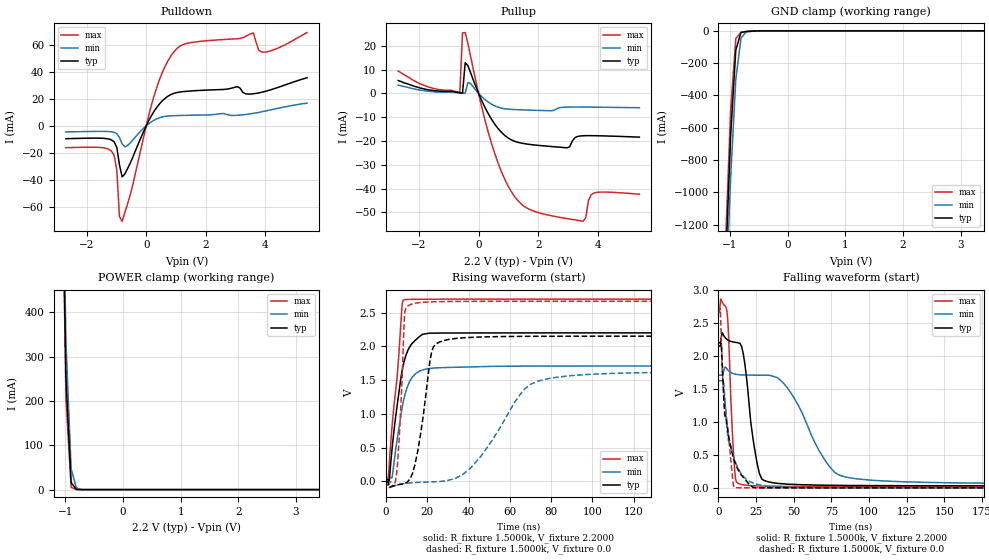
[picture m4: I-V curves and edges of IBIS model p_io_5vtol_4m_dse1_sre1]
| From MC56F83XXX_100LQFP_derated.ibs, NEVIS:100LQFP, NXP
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[Model] p_io_5vtol_4m_dse1_sre1
|   Model p_io_5vtol_4m_dse1_sre1
| Library cells for typ/min/max conditions are connected as defined below:
|  pad - External Pad
|  ipp_do - Core Input
|  ipp_obe - Output Buffer Enable
|  esd_boost - vdd_s_3v
|  esd_bus - vdd_s_3v
|  ipp_ame - vss_s_lv
|  ipp_dse - vdd_s_lv
|  ipp_ina40a_5vtol - NC
|  ipp_ina40b_5vtol - NC
|  ipp_ina_5vtol - NC
|  ipp_ina_mux_3v - NC
|  ipp_ind - NC
|  ipp_ind_3v - NC
|  ipp_pue - vss_s_lv
|  ipp_sre - vdd_s_lv
|  tie_3v - vdd_s_3v
|  tie_hi - vdd_s_lv
|  vbuf_3v - vdd_s_3v
|  vdd_bulk_lv - vdd_s_lv
|  vdd_s_3v - vdd_s_3v
|  vdd_s_lv - vdd_s_lv
|  vss_bulk - vss_s_3v
|  vss_s_3v - vss_s_3v
|  vss_s_lv - vss_s_lv
| All other pins connected to ground
Model_type I/O
Polarity   Non-Inverting
Enable   Active-High
Vinl =   0.7700V
Vinh =   1.5400V
Vmeas =  1.1000V
Cref =   25.0000pF
Rref =   1.0000k
Vref =   0.0V
C_comp   2.5897pF   2.5141pF   2.6932pF
[Temperature Range]   25.0000   0.1250k   -40.0000
[Voltage Range]   2.2000V   1.7100V   2.7000V
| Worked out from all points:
|   slope of the pulldown table from 0 to 0.33 V, typ, clamps not added: 25.7 ohm
|   slope of the pullup table from 0 to 0.33 V, typ, clamps not added: 38.3 ohm
|   GND clamp passes 1 mA (typ) near -0.56 V on its own axis
|   POWER clamp passes 1 mA (typ) near -0.81 V on its own axis
|   rising waveform, R_fixture 1.5000k, V_fixture 2.2000: 20-80 % time 5.84ns typ, 5.78ns min, 4.56ns max; typ from 0.031 V to 2.2 V
|   rising waveform, R_fixture 1.5000k, V_fixture 0.0: 20-80 % time 5.78ns typ, 20.7ns min, 2.31ns max; typ from 0 V to 2.15 V
|   falling waveform, R_fixture 1.5000k, V_fixture 2.2000: 20-80 % time 6.8ns typ, 21.8ns min, 2.96ns max; typ from 2.2 V to 0.031 V
|   falling waveform, R_fixture 1.5000k, V_fixture 0.0: 20-80 % time 7.59ns typ, 8.09ns min, 5.81ns max; typ from 2.15 V to 0 V
[Pulldown]
|Voltage   I(typ)   I(min)   I(max)
-2.7V     -9.58mA    -4.57mA    -16.24mA
-1.17V    -10.45mA   -4.486mA   -18.73mA
-990mV    -15.98mA   -5.899mA   -32.6mA
-900mV    -28.96mA   -8.727mA   -67.1mA
-810mV    -37.86mA   -13.49mA   -70.68mA
270mV     10.92mA    4.186mA    22.64mA
990mV     24.34mA    7.49mA     56.19mA
3.06V     28.9mA     7.71mA     64.33mA
3.6V      23.63mA    9.2mA      68.56mA
3.78V     24.28mA    9.8mA      55.81mA
4.05V     25.71mA    11.1mA     54.67mA
5.4V      35.5mA     16.7mA     68.9mA
[Pullup]
|Voltage   I(typ)   I(min)   I(max)
-2.7V     5.4mA      3.5mA      9.4mA
-630mV    252.5uA    218.2uA    372uA
-540mV    133.6uA    121.1uA    25.42mA
-450mV    12.88mA    56.63uA    25.55mA
-270mV    8.722mA    4.155mA    15.59mA
540mV     -12.86mA   -5.202mA   -25.17mA
990mV     -18.7mA    -6.605mA   -38.86mA
1.44V     -20.88mA   -6.905mA   -46.53mA
2.97V     -22.84mA   -5.75mA    -52.58mA
3.51V     -17.79mA   -5.732mA   -53.71mA
3.87V     -17.76mA   -5.78mA    -41.87mA
5.4V      -18.36mA   -6.02mA    -42.31mA
[GND_clamp]
|Voltage   I(typ)   I(min)   I(max)
-2.7V     -20.35A    -20.38A    -20.37A
-1.08V    -1.486A    -1.737A    -1.339A
-990mV    -654.8mA   -915.7mA   -496.6mA
-900mV    -120.3mA   -300.6mA   -47.98mA
-810mV    -10.43mA   -45.61mA   -9.206mA
-720mV    -3.577mA   -6.172mA   -6.342mA
-540mV    -682.6uA   -563.7uA   -1.265mA
5.4V      0A         0A         0A
[POWER_clamp]
|Voltage   I(typ)   I(min)   I(max)
-2.7V     20.23A     19.96A     20.45A
-1.08V    950.5mA    990.2mA    948mA
-990mV    252.7mA    333.8mA    206.6mA
-900mV    16.05mA    47.59mA    5.278mA
-810mV    508.3uA    3.841mA    61.17uA
-720mV    15.33uA    281.3uA    694.4nA
-630mV    461.8nA    20.43uA    7.955nA
5.4V      0A         0A         0A
[Ramp]
| variable   typ   min   max
dV/dt_r  0.6016/24.4085n   0.2055/56.3670n   1.0880/10.0620n
dV/dt_f  0.7284/40.9818n   0.2179/77.6681n   1.2636/15.3351n
R_load = 50.0000
[Rising Waveform]
R_fixture= 1.5000k
V_fixture= 2.2000
V_fixture_min= 1.7100
V_fixture_max= 2.7000
|time   V(typ)   V(min)   V(max)
0s        31.17mV    60.03mV    18.84mV
899.9ps   31.66mV    60.02mV    -22.79mV
1.51ns    13.16mV    60.44mV    267.9mV
2.898ns   495.8mV    62.89mV    830.2mV
5.303ns   1.116V     615.1mV    1.54V
7.252ns   1.558V     1.004V     2.424V
8.289ns   1.724V     1.181V     2.687V
14.25ns   2.094V     1.596V     2.698V
24.37ns   2.196V     1.682V     2.699V
250ns     2.2V       1.71V      2.7V
[Rising Waveform]
R_fixture= 1.5000k
V_fixture= 0.0
V_fixture_min= 0.0
V_fixture_max= 0.0
|time   V(typ)   V(min)   V(max)
0s        554.5pV    116.9nV    15.42pV
4.607ns   -56.99mV   -58.21mV   18.73mV
6.434ns   -45.92mV   -44.25mV   696mV
8.886ns   -28.72mV   -31.27mV   2.436V
12.57ns   105.7mV    -20.07mV   2.628V
22.09ns   1.925V     -8.013mV   2.66V
27.79ns   2.085V     3.953mV    2.664V
40.95ns   2.133V     198.4mV    2.667V
78.42ns   2.15V      1.521V     2.668V
250ns     2.151V     1.626V     2.668V
[Falling Waveform]
R_fixture= 1.5000k
V_fixture= 2.2000
V_fixture_min= 1.7100
V_fixture_max= 2.7000
|time   V(typ)   V(min)   V(max)
0s        2.2V       1.71V      2.7V
5.586ns   2.253V     1.806V     2.691V
10.58ns   2.21V      1.729V     321.7mV
13.08ns   2.201V     1.719V     68.43mV
17.53ns   1.881V     1.712V     42.81mV
25.7ns    370.6mV    1.71V      29.35mV
31.91ns   98.53mV    1.71V      25.6mV
46.04ns   55.8mV     1.51V      21.78mV
80.6ns    37.23mV    188.8mV    19.29mV
250ns     31.22mV    63.37mV    18.84mV
[Falling Waveform]
R_fixture= 1.5000k
V_fixture= 0.0
V_fixture_min= 0.0
V_fixture_max= 0.0
|time   V(typ)   V(min)   V(max)
0s        2.151V     1.626V     2.668V
1.232ns   2.151V     1.626V     2.692V
2.001ns   2.125V     1.626V     2.105V
3.213ns   1.464V     1.635V     1.524V
4.117ns   1.127V     1.391V     1.345V
6.31ns    851mV      756.6mV    860.5mV
9.298ns   506.8mV    538.7mV    148.7mV
10.7ns    402mV      428mV      1.999mV
25.49ns   1.395mV    54.99mV    445.4uV
250ns     -45.38uV   6.424uV    1.035uV
